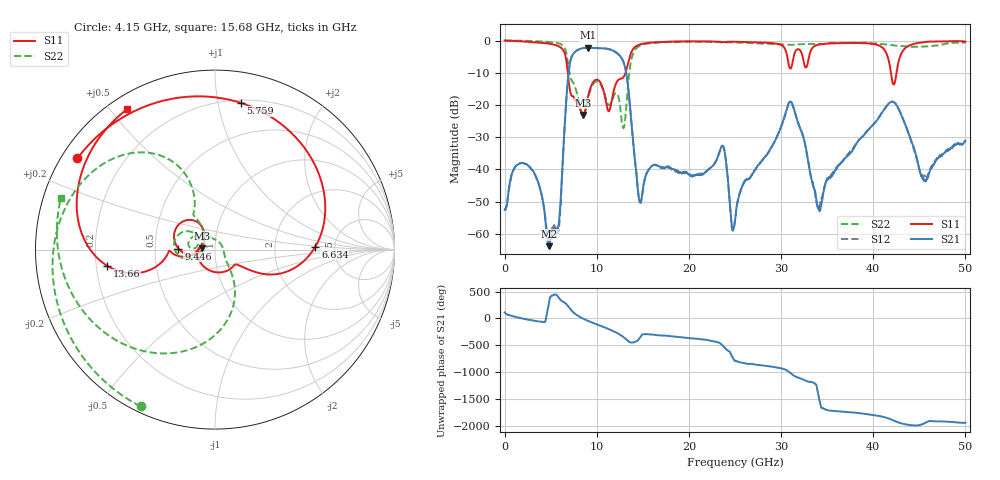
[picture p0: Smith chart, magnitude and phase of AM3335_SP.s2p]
!Keysight Technologies,N5245B,MY58422270,A.16.20.02
!Date: Friday, January 23, 2026 00:55:46
!Correction: S11(C  2-Port  )
!S21(C  2-Port  )
!S12(C  2-Port  )
!S22(C  2-Port  )
!S2P File: Measurements: S11, S21, S12, S22:
# Hz S  dB  R 50
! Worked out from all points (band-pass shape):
!   3201 points, 10 MHz to 50 GHz, reference 50 ohm
!   highest |S21| = -2.21 dB at 9.055 GHz (marker M1); lowest = -63.8 dB at 4.868 GHz (marker M2)
!   |S21| within 3 dB of the highest: 7.259 GHz to 12.65 GHz (5.389 GHz wide, 54.1 % of centre)
!   lowest |S11| = -23.1 dB at 8.508 GHz (marker M3), VSWR 1.15, Z = 43.5 + j0.641 ohm
!   |S11| at or under -10 dB: 6.858 GHz to 13.13 GHz (6.27 GHz wide, 62.7 % of centre); 41.92 GHz to 42.53 GHz (609.4 MHz wide, 1.44 % of centre)
!   |S22| runs from -27.2 to 0.0 dB; largest |S21 - S12| = 0.0056
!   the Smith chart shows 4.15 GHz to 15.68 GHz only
!   S11 on the Smith chart (normalised r, x): 4.15 GHz: 0.05, +0.30; 5.759 GHz: 0.22, +1.17; 6.634 GHz: 3.53, +0.17; 9.446 GHz: 0.66, +0.01; 13.66 GHz: 0.24, -0.07; 15.68 GHz: 0.05, +0.55
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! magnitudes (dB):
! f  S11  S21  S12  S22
! 10 MHz  0.0  -52.5  -52.5  0.0
! 1.76 GHz  -0.2  -38.1  -38.0  0.0
! 4.15 GHz  -0.7  -49.6  -49.5  -0.3
! 4.868 GHz  -1.0  -63.8  -62.4  -0.4
! 5.759 GHz  -1.6  -58.6  -60.1  -0.8
! 6.634 GHz  -5.0  -21.4  -21.4  -3.1
! 8.352 GHz  -22.5  -2.5  -2.5  -22.1
! 8.508 GHz  -23.1  -2.4  -2.4  -23.3
! 9.055 GHz  -17.5  -2.2  -2.2  -18.2
! 9.446 GHz  -13.8  -2.2  -2.2  -14.4
! 12.9 GHz  -11.4  -6.6  -6.6  -27.2
! 13.66 GHz  -4.3  -22.1  -22.1  -7.3
! 14.65 GHz  -1.3  -49.9  -49.8  -1.7
! 15.68 GHz  -0.7  -39.9  -39.8  -0.9
! 16.68 GHz  -0.5  -38.9  -39.1  -0.6
! 23.65 GHz  -0.5  -32.6  -32.7  -0.6
! 25 GHz  -0.4  -56.2  -56.0  -0.6
! 30.96 GHz  -8.6  -19.0  -19.0  -1.4
! 33.35 GHz  -2.5  -43.5  -43.6  -1.1
! 41.67 GHz  -6.1  -19.6  -19.6  -1.3
! 45.55 GHz  -0.4  -43.1  -41.9  -1.9
! 50 GHz  -0.3  -31.0  -31.3  -0.6
